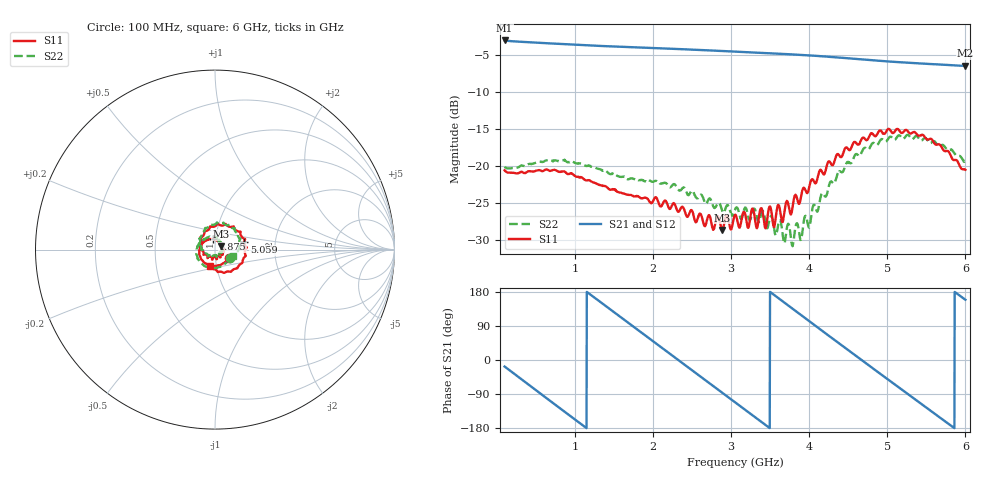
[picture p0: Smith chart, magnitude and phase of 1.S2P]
!Agilent Technologies,E5071C,MY46316741,A.11.02
!Date: Thu Dec 16 09:43:42 2021
!Data & Calibration Information:
!Freq	S11:SOLT4(ON)	S21:SOLT4(ON)	S12:SOLT4(ON)	S22:SOLT4(ON)
!PortZ  Port1:50+j0  Port2:50+j0
!Above PortZ is port z conversion or system Z0 setting when saving the data.
!When reading, reference impedance value at option line is always used.
# Hz S dB R 50
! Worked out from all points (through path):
!   1593 points, 100 MHz to 6 GHz, reference 50 ohm
!   highest |S21| = -3.01 dB at 100 MHz (marker M1); lowest = -6.4 dB at 6 GHz (marker M2)
!   group delay of S21, straight-line fit = 426 ps
!   lowest |S11| = -28.7 dB at 2.883 GHz (marker M3), VSWR 1.08, Z = 53.3 + j1.93 ohm
!   |S11| at or under -10 dB: start of sweep to end of sweep
!   |S22| runs from -30.9 to -15.8 dB; largest |S21 - S12| = 0.004
!   S11 on the Smith chart (normalised r, x): 100 MHz: 1.17, -0.11; 1.875 GHz: 0.97, +0.12; 5.059 GHz: 1.38, +0.12; 6 GHz: 0.93, -0.17
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1e8  -20.61 -30.4  -3.01 -17.3  -3.02 -17.3  -20.13 -28.9
3.631281e8  -20.98 -80.5  -3.23 -58.2  -3.23 -58.1  -20.03 -77.1
5.817839e8  -20.73 -120.0  -3.36 -92.2  -3.36 -92.2  -19.49 -114.2
8.078518e8  -20.83 -156.2  -3.48 -127.2  -3.49 -127.1  -19.35 -147.3
1.085804e9  -21.56 167.5  -3.63 -170.1  -3.64 -170.1  -19.69 -179.6
1.530528e9  -23.40 125.5  -3.84 121.7  -3.85 121.7  -21.29 145.0
1.875188e9  -24.39 99.8  -3.99 68.8  -4.00 68.8  -22.01 124.6
2.067902e9  -24.89 90.1  -4.07 39.3  -4.08 39.3  -22.21 111.8
2.442211e9  -26.93 54.9  -4.23 -18.3  -4.24 -18.2  -23.90 85.2
2.883229e9  -28.70 29.6  -4.44 -85.9  -4.46 -85.8  -26.00 64.1
3.05e9  -26.67 13.4  -4.53 -111.5  -4.54 -111.3  -25.96 48.8
3.305716e9  -27.21 -10.1  -4.66 -150.6  -4.66 -150.5  -25.90 35.2
3.528078e9  -27.12 -52.8  -4.76 175.2  -4.76 175.4  -27.11 1.3
3.7875e9  -25.56 -131.1  -4.91 135.2  -4.91 135.4  -30.89 -63.1
4.035804e9  -21.82 -178.5  -5.07 97.1  -5.07 97.3  -26.13 -136.8
4.27299e9  -19.59 139.4  -5.25 60.7  -5.25 60.8  -22.15 179.8
4.554648e9  -17.13 85.6  -5.48 17.6  -5.48 17.7  -19.35 134.0
5.017902e9  -14.99 19.3  -5.86 -52.7  -5.86 -52.5  -16.24 73.4
5.058668e9  -15.49 14.8  -5.89 -58.9  -5.90 -58.6  -16.16 72.0
5.440389e9  -15.83 -39.1  -6.14 -116.5  -6.13 -116.3  -16.57 27.2
5.725754e9  -17.95 -76.1  -6.31 -159.8  -6.29 -159.3  -17.30 1.4
6e9  -20.54 -106.9  -6.44 159.0  -6.43 159.3  -19.42 -20.9
